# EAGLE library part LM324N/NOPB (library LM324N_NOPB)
Check availability
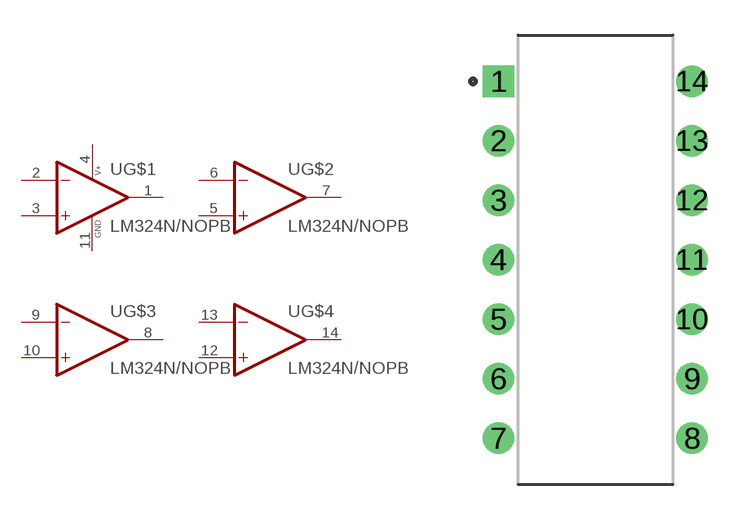
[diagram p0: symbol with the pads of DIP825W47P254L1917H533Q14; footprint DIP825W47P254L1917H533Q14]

Designator prefix -; gates G$1=LM324N/NOPB_SECTION1 G$2=LM324N/NOPB_SECTION2 G$3=LM324N/NOPB_SECTION3 G$4=LM324N/NOPB_SECTION4

## LM324N/NOPB (Availability: In Stock; Description: Quad, 30-V, 1.2-MHz operational amplifier; MF: Texas Instruments; MP: LM324N; Package: PDIP-14 Texas Instruments; Price: None; Purchase-URL: https://pricing.snapeda.com/search/part/LM324N/?ref=eda)  [DIP825W47P254L1917H533Q14]
1  G$1:1OUT  out
2  G$1:1IN-  in
3  G$1:1IN+  in
4  G$1:V+  pwr
5  G$2:2IN+  in
6  G$2:2IN-  in
7  G$2:2OUT  out
8  G$3:3OUT  out
9  G$3:3IN-  in
10  G$3:3IN+  in
11  G$1:GND  pwr
12  G$4:4IN+  in
13  G$4:4IN-  in
14  G$4:4OUT  out

## Footprint DIP825W47P254L1917H533Q14 (pad centres in mm)
drill 0.83 pad 1.18 square: 1 -4.128,7.62
drill 0.83 pad 1.18: 2 -4.128,5.08; 3 -4.128,2.54; 4 -4.128,0; 5 -4.128,-2.54; 6 -4.128,-5.08; 7 -4.128,-7.62; 8 4.128,-7.62; 9 4.128,-5.08; 10 4.128,-2.54; 11 4.128,0; 12 4.128,2.54; 13 4.128,5.08; 14 4.128,7.62

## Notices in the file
This work is licensed under a Creative Commons Attribution-ShareAlike 4.0 International License (CC BY-SA) with Design Exception 1.0
